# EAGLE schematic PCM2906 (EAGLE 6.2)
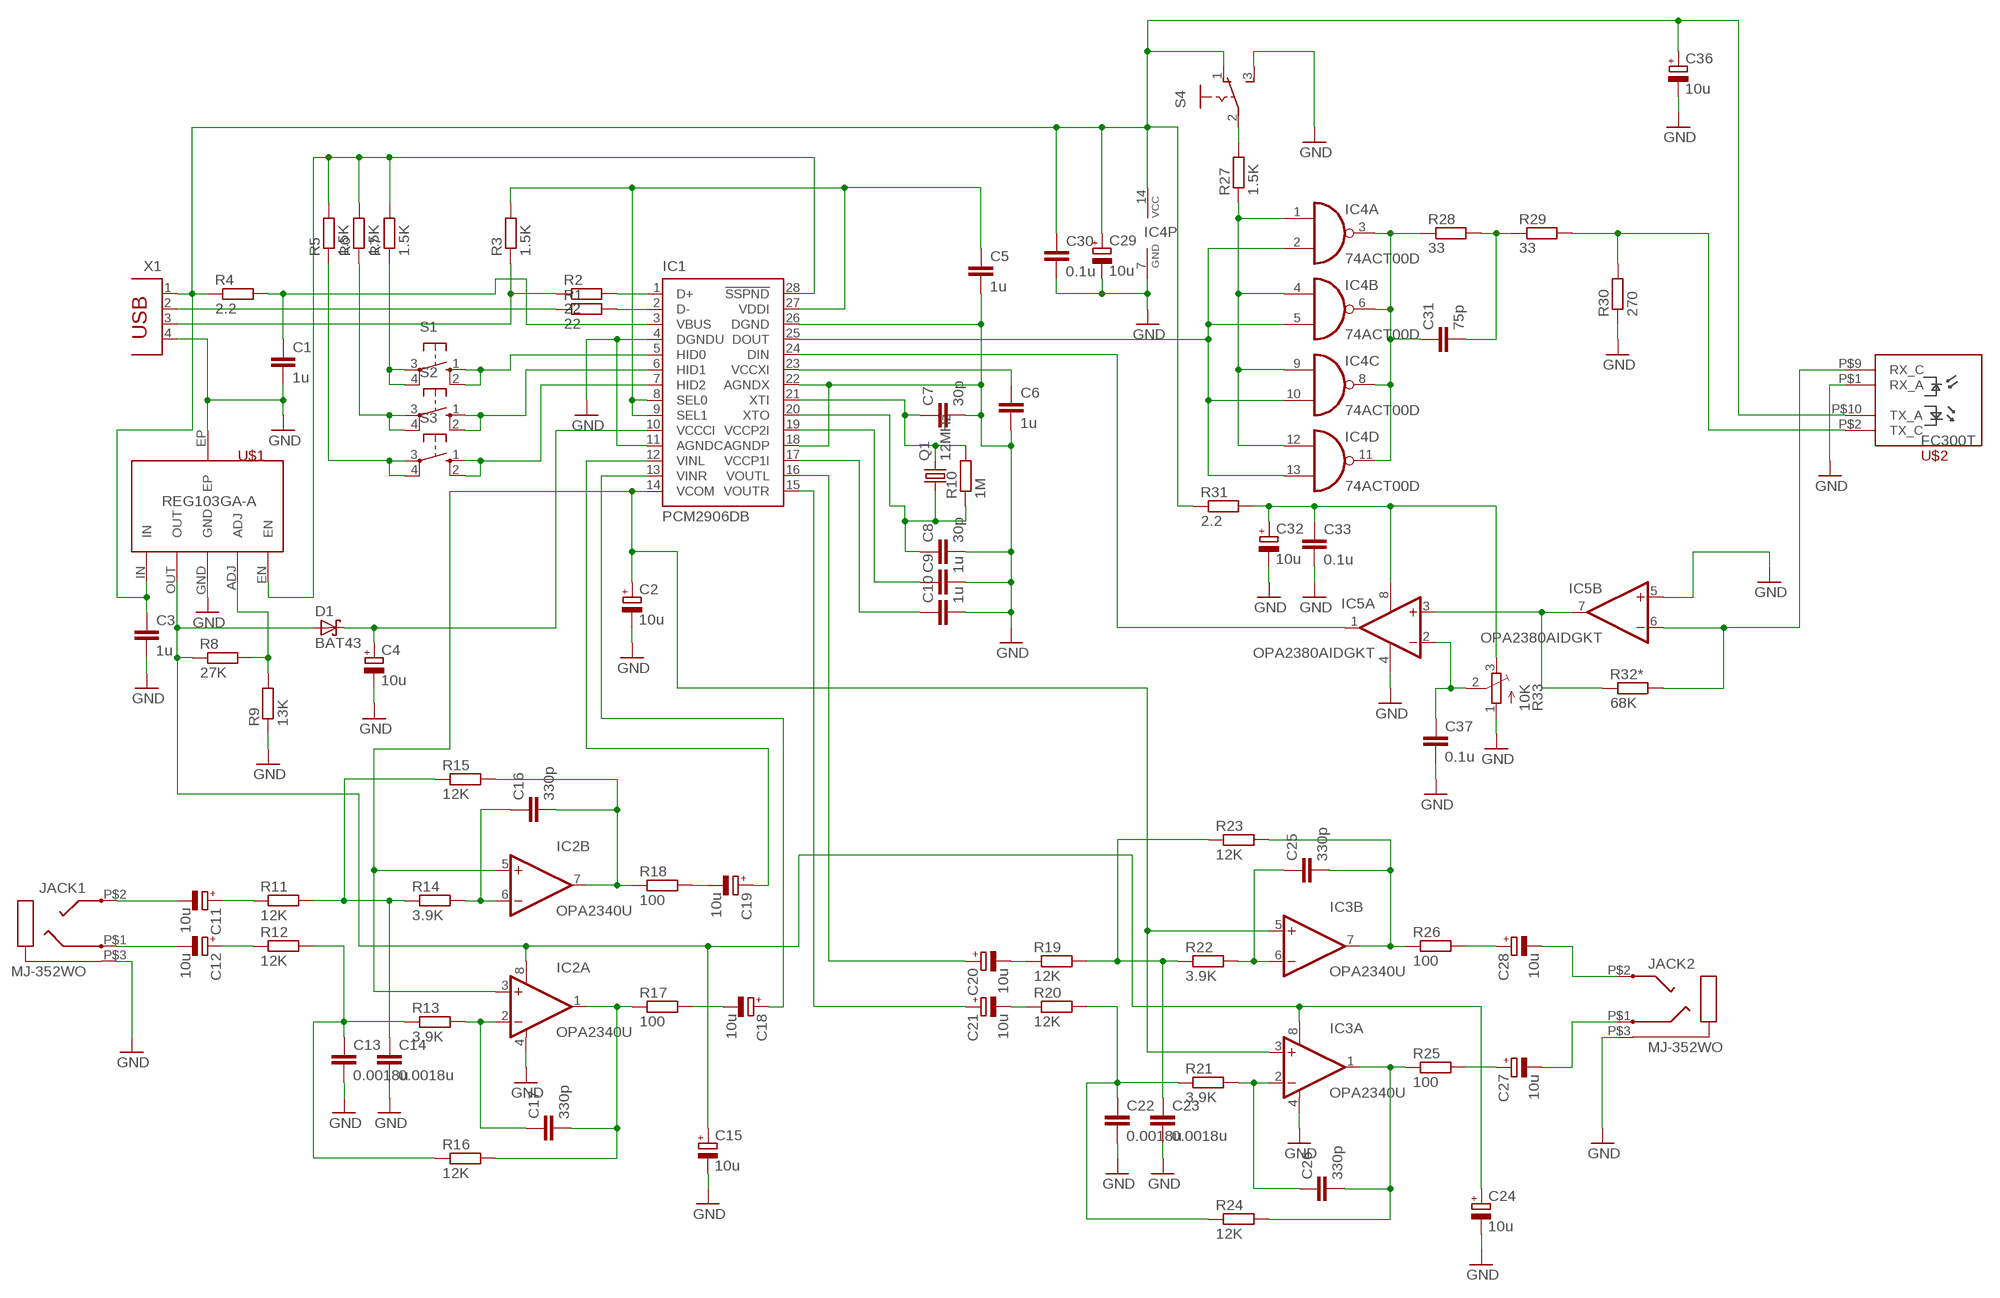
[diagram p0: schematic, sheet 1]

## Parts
C1  1u  C-EUC2012  [C2012]
C2  10u  CPOL-EU085CS-1AR  [085CS_1AR]
C3  1u  C-EUC2012  [C2012]
C4  10u  CPOL-EU085CS-1AR  [085CS_1AR]
C5  1u  C-EUC2012  [C2012]
C6  1u  C-EUC2012  [C2012]
C7  30p  C-EUC2012  [C2012]
C8  30p  C-EUC2012  [C2012]
C9  1u  C-EUC2012  [C2012]
C10  1u  C-EUC2012  [C2012]
C11  10u  CPOL-EU085CS-1AR  [085CS_1AR]
C12  10u  CPOL-EU085CS-1AR  [085CS_1AR]
C13  0.0018u  C-EUC2012  [C2012]
C14  0.0018u  C-EUC2012  [C2012]
C15  10u  CPOL-EU085CS-1AR  [085CS_1AR]
C16  330p  C-EUC2012  [C2012]
C17  330p  C-EUC2012  [C2012]
C18  10u  CPOL-EU085CS-1AR  [085CS_1AR]
C19  10u  CPOL-EU085CS-1AR  [085CS_1AR]
C20  10u  CPOL-EU085CS-1AR  [085CS_1AR]
C21  10u  CPOL-EU085CS-1AR  [085CS_1AR]
C22  0.0018u  C-EUC2012  [C2012]
C23  0.0018u  C-EUC2012  [C2012]
C24  10u  CPOL-EU085CS-1AR  [085CS_1AR]
C25  330p  C-EUC2012  [C2012]
C26  330p  C-EUC2012  [C2012]
C27  10u  CPOL-EU085CS-1AR  [085CS_1AR]
C28  10u  CPOL-EU085CS-1AR  [085CS_1AR]
C29  10u  CPOL-EU085CS-1AR  [085CS_1AR]
C30  0.1u  C-EUC2012  [C2012]
C31  75p  C-EUC2012  [C2012]
C32  10u  CPOL-EU085CS-1AR  [085CS_1AR]
C33  0.1u  C-EUC2012  [C2012]
C36  10u  CPOL-EU085CS-1AR  [085CS_1AR]
C37  0.1u  C-EUC2012  [C2012]
D1  BAT43  SCHOTTKY-DIODESMD  [SMB]
IC1  PCM2906DB  [SSOP28DB]
IC2  OPA2340U  [SO08]
IC3  OPA2340U  [SO08]
IC4  74ACT00D  [SO14]
IC5  OPA2380AIDGKT  OPA2344E  [MSOP08]
JACK1  MJ-352WO  [MJ-352]
JACK2  MJ-352WO  [MJ-352]
Q1  12MHz  CRYSTALHC49S  [HC49/S]
R1  22  R-EU_R2012  [R2012]
R2  22  R-EU_R2012  [R2012]
R3  1.5K  R-EU_R2012  [R2012]
R4  2.2  R-EU_R2012  [R2012]
R5  1.5K  R-EU_R2012  [R2012]
R6  1.5K  R-EU_R2012  [R2012]
R7  1.5K  R-EU_R2012  [R2012]
R8  27K  R-EU_R2012  [R2012]
R9  13K  R-EU_R2012  [R2012]
R10  1M  R-EU_R2012  [R2012]
R11  12K  R-EU_R2012  [R2012]
R12  12K  R-EU_R2012  [R2012]
R13  3.9K  R-EU_R2012  [R2012]
R14  3.9K  R-EU_R2012  [R2012]
R15  12K  R-EU_R2012  [R2012]
R16  12K  R-EU_R2012  [R2012]
R17  100  R-EU_R2012  [R2012]
R18  100  R-EU_R2012  [R2012]
R19  12K  R-EU_R2012  [R2012]
R20  12K  R-EU_R2012  [R2012]
R21  3.9K  R-EU_R2012  [R2012]
R22  3.9K  R-EU_R2012  [R2012]
R23  12K  R-EU_R2012  [R2012]
R24  12K  R-EU_R2012  [R2012]
R25  100  R-EU_R2012  [R2012]
R26  100  R-EU_R2012  [R2012]
R27  1.5K  R-EU_R2012  [R2012]
R28  33  R-EU_R2012  [R2012]
R29  33  R-EU_R2012  [R2012]
R30  270  R-EU_R2012  [R2012]
R31  2.2  R-EU_R2012  [R2012]
R32*  68K  R-EU_R2012  [R2012]
R33  10K  TRIM_EU-3223W  [3223W]
S1  10-XX  [B3F-10XX]
S2  10-XX  [B3F-10XX]
S3  10-XX  [B3F-10XX]
S4  255SB  [255SB]
U$1  REG103GA-A  [REG103GA-A]
U$2  FC300T  [FC300T]
X1  PN61729  [PN61729]

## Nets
GND: C1.2 C2.- C3.2 C4.- C5.2 C6.2 C7.2 C8.2 C9.2 C10.2 C13.2 C14.2 C15.- C22.2 C23.2 C24.- C29.- C30.2 C32.- C33.2 C36.- C37.2 IC1.4(DGNDU) IC1.11(AGNDC) IC1.18(AGNDP) IC1.22(AGNDX) IC1.26(DGND) IC2.4(A:V-) IC3.4(A:V-) IC4.7(P:GND) IC5.4(A:V-) IC5.5(B:+IN) JACK1.P$3(G) JACK2.P$3(G) R9.1 R30.1 R33.1(A) S4.3(S) U$1.EP U$1.GND U$2.P$1(RX_A) X1.4
N$1: IC1.1(D+) R2.2
N$2: IC1.2(D-) R1.2
N$3: R1.1 X1.2
N$4: R2.1 R3.1 X1.3
N$5: C5.1 IC1.8(SEL0) IC1.9(SEL1) IC1.27(VDDI) R3.2
N$6: C3.1 C29.+ C30.1 C36.+ IC4.14(P:VCC) R4.1 R31.1 S4.1(O) U$1.IN U$2.P$10(TX_A) X1.1
N$7: C1.1 IC1.3(VBUS) R4.2
N$8: C17.2 IC2.1(A:OUT) R16.2 R17.1
N$9: IC1.5(HID0) S1.1(S) S1.2(S1)
N$10: R7.1 S1.3(P) S1.4(P1)
N$11: IC1.6(HID1) S2.1(S) S2.2(S1)
N$12: IC1.7(HID2) S3.1(S) S3.2(S1)
N$13: IC1.28(!SSPND) R5.2 R6.2 R7.2 U$1.EN
N$14: R5.1 S3.3(P) S3.4(P1)
N$15: R6.1 S2.3(P) S2.4(P1)
N$16: C17.1 IC2.2(A:-IN) R13.2
N$17: R8.2 R9.2 U$1.ADJ
N$18: C4.+ D1.C IC1.10(VCCCI)
N$19: C6.1 IC1.23(VCCXI)
N$20: C7.1 IC1.21(XTI) Q1.2 R10.2
N$21: C8.1 IC1.20(XTO) Q1.1 R10.1
N$22: C11.+ R11.1
N$23: C9.1 IC1.19(VCCP2I)
N$24: C11.- JACK1.P$2(L)
N$25: C10.1 IC1.17(VCCP1I)
N$26: C12.- JACK1.P$1(R)
N$27: C12.+ R12.1
N$28: C13.1 R12.2 R13.1 R16.1
N$29: C15.+ C24.+ D1.A IC2.8(A:V+) IC3.8(A:V+) R8.1 U$1.OUT
N$30: C14.1 R11.2 R14.1 R15.1
N$31: C16.1 IC2.6(B:-IN) R14.2
N$32: C20.- R19.1
N$33: C21.- R20.1
N$34: C16.2 IC2.7(B:OUT) R15.2 R18.1
N$35: C28.+ R26.2
N$36: C27.+ R25.2
N$37: C21.+ IC1.15(VOUTR)
N$38: C20.+ IC1.16(VOUTL)
N$39: C18.- R17.2
N$40: C18.+ IC1.13(VINR)
N$41: C19.- R18.2
N$42: C19.+ IC1.12(VINL)
N$43: C31.1 IC4.3(A:O) IC4.6(B:O) IC4.8(C:O) IC4.11(D:O) R28.1
N$44: C27.- JACK2.P$1(R)
N$45: C28.- JACK2.P$2(L)
N$46: IC4.1(A:I0) IC4.4(B:I0) IC4.9(C:I0) IC4.12(D:I0) R27.1
N$47: C22.1 R20.2 R21.1 R24.1
N$48: C23.1 R19.2 R22.1 R23.1
N$49: C31.2 R28.2 R29.1
N$50: C26.1 IC3.2(A:-IN) R21.2
N$51: C25.1 IC3.6(B:-IN) R22.2
N$52: C2.+ IC1.14(VCOM) IC2.3(A:+IN) IC2.5(B:+IN) IC3.3(A:+IN) IC3.5(B:+IN)
N$53: C26.2 IC3.1(A:OUT) R24.2 R25.1
N$54: C25.2 IC3.7(B:OUT) R23.2 R26.1
N$55: R29.2 R30.2 U$2.P$2(TX_C)
N$56: IC1.25(DOUT) IC4.2(A:I1) IC4.5(B:I1) IC4.10(C:I1) IC4.13(D:I1)
N$57: R27.2 S4.2(P)
N$59: IC5.6(B:-IN) R32*.2 U$2.P$9(RX_C)
N$60: C32.+ C33.1 IC5.8(A:V+) R31.2 R33.3(E)
N$61: IC1.24(DIN) IC5.1(A:OUT)
N$63: IC5.3(A:+IN) IC5.7(B:OUT) R32*.1
N$67: C37.1 IC5.2(A:-IN) R33.2(S)

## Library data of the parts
C1 C3 C5-C10 C13 C14 C16 C17 C22 C23 C25 C26 C30 C31 C33 C37 = rcl:C-EU: CAPACITOR, European symbol
C2 C4 C11 C12 C15 C18-C21 C24 C27-C29 C32 C36 = rcl:CPOL-EU: POLARIZED CAPACITOR, European symbol
D1 = diode:SCHOTTKY-DIODE: Schottky Diode
IC1 = texas:PCM290*: STEREO AUDIO CODEC WITH USB INTERFACE SINGLE-ENDED ANALOG INPUT/OUTPUT AND S/PDIF
IC2 IC3 = burr-brown:OPA2340: Single-Supply, Rail-to-Rail Operational Amplifiers MicroAmplifier(TM) Series; Product Folder:OPA2340
IC4 = 74xx-eu:74*00: Quad 2-input NAND gate
IC5 = linear:OPA2*: Dual Operational Amplifier Low Power, Single-Supply, Rail-To-Rail Operational Amplifier Source: http://focus.ti.com/lit/ds/symlink/opa2345.pdf http://focus.ti.com .. opa241.pdf http://focus.ti.com/lit/ds/symlink/opa2134.pdf
JACK1 JACK2 = my_lib:MJ-352
Q1 = crystal:CRYSTAL: CRYSTAL
R1-R31 R32* = rcl:R-EU_: RESISTOR, European symbol
R33 = pot:TRIM_EU-: POTENTIOMETER
S1-S3 = switch-omron:10-XX: OMRON SWITCH
S4 = switch:255SB: SLIDING SWITCH Distributor Buerklin, 11G810
U$1 = My-custom:REG103GA-A: Single Output LDO, 500mA, Adj.(1.295 to 5.5V), Low Noise, Fast Transient Response
U$2 = Firecomms:FC300T: Firecomms Optolock having LED and PIN phtodiode
X1 = con-berg:PN61729: BERG USB connector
